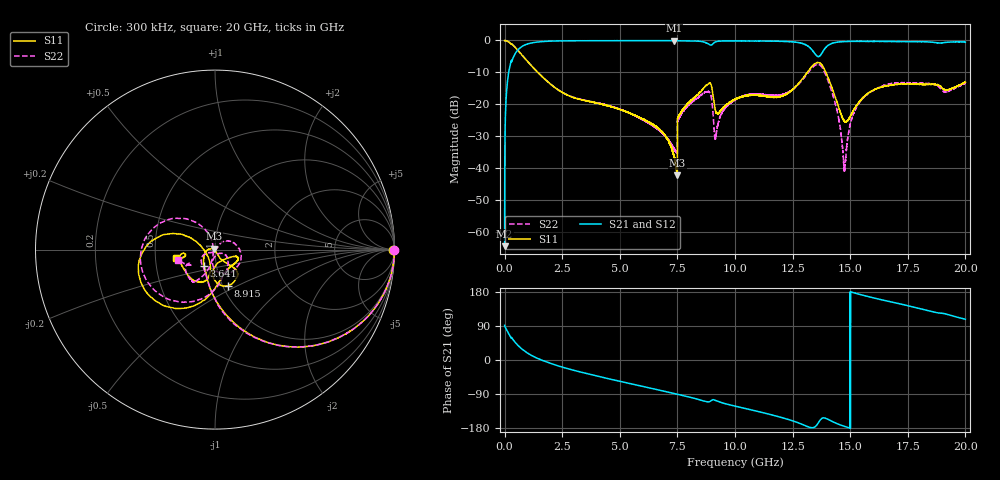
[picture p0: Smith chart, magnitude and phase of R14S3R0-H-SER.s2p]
!{R14S3R0}
!Johanson Technology Inc.
!www.johansontechnology.com
!Test Board Conditions:
!Substrate Type  RO4350B
!Substrate Thickness  20 mil
!Substrate Dk  3.66
!TL Type: GCPW
!TL Trace Width  36 mil
!TL Gap  12 mil
!Electrode orientation  Horizontal
!DUT TOPOLOGY	SERIES
!Mounting Pad LxW  26x36 mil
! Created Wed Nov 25 17:33:21 2020
! 2 Port Network Data from SP1.SP block
! freq  magS11  angS11  magS21  angS21  magS12  angS12  magS22  angS22
# khz S ma R 50
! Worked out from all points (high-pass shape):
!   20001 points, 300 kHz to 20 GHz, reference 50 ohm
!   highest |S21| = -0.05 dB at 7.358 GHz (marker M1); lowest = -64.5 dB at 300 kHz (marker M2)
!   |S21| within 3 dB of the highest: 567 MHz to 13.35 GHz (12.78 GHz wide, 184 % of centre); 13.85 GHz to end of sweep
!   lowest |S11| = -42.3 dB at 7.498 GHz (marker M3), VSWR 1.02, Z = 49.4 + j0.499 ohm
!   |S11| at or under -10 dB: 1.439 GHz to 13.14 GHz (11.7 GHz wide, 161 % of centre); 13.94 GHz to end of sweep
!   |S22| runs from -41.0 to 0.0 dB; largest |S21 - S12| = 0.018
!   S11 on the Smith chart (normalised r, x): 300 kHz: open; 3.641 GHz: 0.87, -0.16; 8.915 GHz: 1.05, -0.44; 20 GHz: 0.64, -0.06
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300  0.9919 -0.2  0.0005967 91.5  0.0006058 89.6  0.9974 -0.1
127300  0.9713 -14.8  0.2319 75.1  0.233 75.0  0.9721 -14.8
446300  0.7876 -42.1  0.6105 47.6  0.6116 47.7  0.788 -42.0
1373300  0.3339 -83.6  0.9391 5.8  0.9386 5.7  0.3354 -84.3
3334300  0.1177 -119.5  0.9892 -32.3  0.9897 -32.3  0.1188 -123.3
3641300  0.111 -123.2  0.9899 -37.0  0.9901 -37.0  0.1123 -129.0
6667300  0.04164 -177.1  0.9925 -78.9  0.9927 -78.9  0.03996 -152.2
7358300  0.015 159.6  0.9944 -88.4  0.993 -88.5  0.01999 -127.5
7498300  0.007702 139.0  0.9926 -90.4  0.9919 -90.4  0.01731 -106.3
7600300  0.0691 -55.3  0.9888 -91.9  0.9895 -91.8  0.06343 44.4
8915300  0.2125 -70.9  0.8525 -109.5  0.8534 -109.5  0.1514 -62.6
9173300  0.07552 -75.7  0.956 -107.2  0.9573 -107.3  0.03216 -42.8
1.00003e7  0.1199 -18.2  0.9817 -121.6  0.9817 -121.7  0.1172 -52.3
1.21193e7  0.1388 -65.3  0.9664 -153.5  0.9702 -153.4  0.1451 -72.0
1.33343e7  0.3905 -122.8  0.716 -178.7  0.7182 -179.0  0.3669 -129.1
1.36683e7  0.4455 -162.2  0.5657 -161.1  0.5647 -161.6  0.4148 -176.8
1.40723e7  0.2453 158.6  0.8532 -157.7  0.8494 -157.8  0.2157 129.9
1.44643e7  0.09807 160.1  0.9421 -168.8  0.9409 -168.8  0.06887 110.9
1.47543e7  0.05411 -160.9  0.9617 -175.2  0.9611 -175.2  0.009129 -169.0
1.53213e7  0.1005 -104.8  0.9685 174.6  0.9703 174.5  0.09634 -107.5
1.66673e7  0.1944 -113.3  0.9662 154.7  0.9595 154.6  0.2076 -121.2
2e7  0.2225 -168.1  0.9447 107.4  0.9453 107.6  0.2139 -164.9
